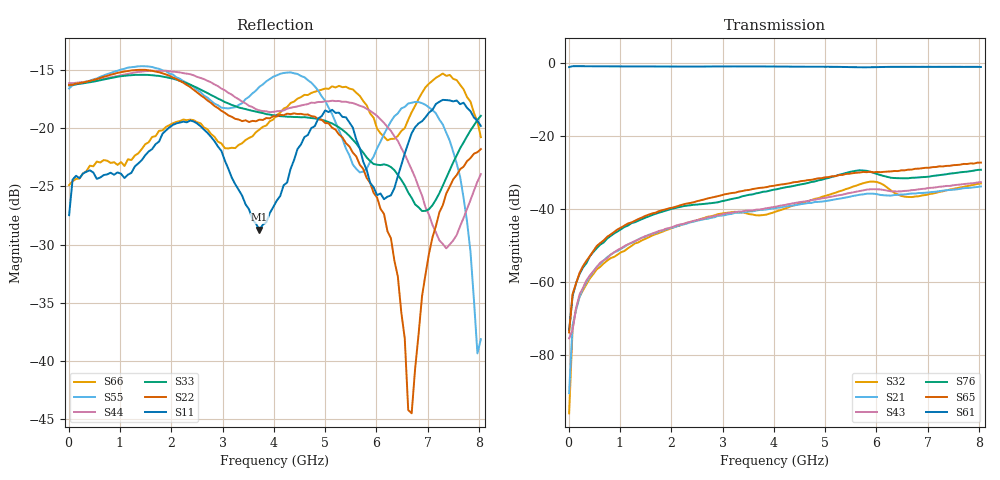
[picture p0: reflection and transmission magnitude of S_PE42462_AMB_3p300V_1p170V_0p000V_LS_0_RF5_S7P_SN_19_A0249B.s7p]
! Device ID: PE42462
! File Path: z:\PE42462\DataSheet S-parameter-6T\AMB\3p300\LS_0_RF5\PE42462_AMB_3p300V_1p170V_0p000V_LS_0_RF5_S7P_SN_19_A0249B.s7p
! Serial: 19
! Lot: A0249B
! Temp: AMB
! VDD: 3.300
! VSS: 0.000
! Control_Hi: 1.170
! Control_Lo: 0.000
! Logic State: LS_0_RF5
! Port 1:
! Port 2:
! Port 3:
! Port 4:
! Port 5:
! Port 6:
! Port 7:
! ThroughPath:1-6
! IDD: 0.0001068498
! ISS/IDD2: -3.1e-008
! IDMM3/IDD3: -2.18e-007
! Comment:
#  Hz  S  RI  R  50
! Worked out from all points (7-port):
!   120 points, 10 MHz to 8.037 GHz, reference 50 ohm
!   strongest paths, dB at 10 MHz, 2.034 GHz, 4.057 GHz, 6.08 GHz, 8.037 GHz:
!     S61: -1.1, -0.9, -0.9, -1.1, -1.0
!     S65: -73.8, -39.5, -33.4, -29.9, -27.2
!     S76: -73.2, -39.8, -34.5, -30.7, -29.2
!     S43: -75.4, -44.8, -39.3, -34.6, -32.6
!     S21: -90.4, -45.0, -39.6, -36.1, -33.8
!     S32: -95.9, -45.1, -40.6, -32.9, -33.0
!   lowest |S11| = -28.7 dB at 3.72 GHz (marker M1), VSWR 1.08, Z = 53.8 + j0.0432 ohm
!   |S11| at or under -10 dB: start of sweep to end of sweep
